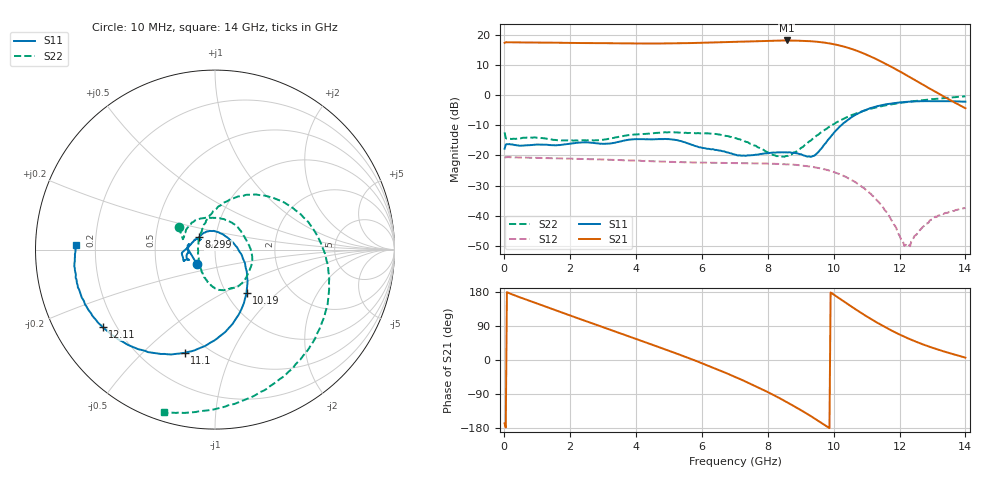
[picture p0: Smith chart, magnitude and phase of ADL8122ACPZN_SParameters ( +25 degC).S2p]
! "Analog Devices, Inc."
! Device:	ADL8122ACPZN
! Description:	"10 kHz to 10 GHz, Wideband, Low Noise Amplifier"
! Conditions:	Vdd = 5.0 V
!		IDQ = 95 mA
!		Pin = -25 dBm
!		Operating Temperature = +25 C (at package bottom)
! Product validation unit SN1 soldered down to Evaluation Board as shown on ADL8122-EVALZ User Guide. Board loss de-embedded from S21 magnitude.  All other RF measurements reference to RF coaxial connector.
! Frequency (GHz)	S11_Mag (dB)	S11_Phase (deg)	S21_Mag (dB)	S21_Phase (deg)	S12_Mag (dB)	S12_Phase (deg)	S22_Mag (dB)	S22_Phase (deg)
#  GHZ  S  DB  R 50
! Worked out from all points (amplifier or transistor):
!   401 points, 10 MHz to 14 GHz, reference 50 ohm
!   highest |S21| = 18.0 dB at 8.579 GHz (marker M1)
!   |S21| within 3 dB of that: start of sweep to 10.6 GHz
!   unconditionally stable (mu >= 1): start of sweep to end of sweep
!   at 2.318 GHz: K = 1.09, MAG = 17.4 dB, |S12| = -21.2 dB
!   at 7.005 GHz: K = 1.12, MAG = 17.9 dB, |S12| = -22.6 dB
!   at 14 GHz: K = 2.02, MAG = 10.7 dB, |S12| = -37.4 dB
!   S11 on the Smith chart (normalised r, x): 10 MHz: 0.81, -0.13; 8.299 GHz: 0.83, +0.12; 10.19 GHz: 1.23, -0.66; 11.1 GHz: 0.38, -0.68; 12.11 GHz: 0.15, -0.31; 14 GHz: 0.13, +0.02
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0.01  -17.82 -141.9  17.25 -167.4  -20.81 12.6  -12.40 147.7
0.184875  -16.37 170.2  17.44 175.0  -20.63 -3.8  -14.54 159.7
1.024275  -16.43 178.5  17.35 148.0  -20.84 -24.8  -14.12 125.2
1.6888  -16.59 -173.4  17.27 127.1  -21.00 -40.9  -15.00 93.4
2.353325  -15.73 -166.2  17.19 106.4  -21.19 -57.1  -15.05 54.8
3.472525  -15.53 -160.6  17.09 71.9  -21.54 -85.5  -13.88 -3.1
4.69665  -14.64 -170.0  17.04 33.9  -22.02 -118.2  -12.53 -46.3
5.920775  -17.33 166.5  17.25 -5.7  -22.38 -152.4  -12.70 -72.8
6.4454  -18.21 152.1  17.41 -23.9  -22.50 -167.8  -12.99 -85.0
7.005  -19.78 145.9  17.60 -44.5  -22.57 175.2  -14.26 -99.4
7.7045  -19.75 148.0  17.84 -72.1  -22.67 152.7  -17.36 -124.6
8.299075  -19.01 141.5  18.01 -98.0  -22.84 132.0  -20.27 -166.6
8.578875  -19.05 129.0  18.04 -111.1  -23.00 121.4  -20.20 164.4
9.348325  -20.34 45.4  17.75 -150.3  -23.83 89.7  -14.65 100.4
9.768025  -15.81 -17.2  17.25 -173.8  -24.75 70.2  -11.34 77.9
10.18772  -10.45 -54.2  16.36 161.7  -26.27 49.4  -8.49 54.6
10.6424  -6.70 -82.9  14.88 135.2  -28.79 26.2  -6.29 29.6
11.09707  -4.44 -106.4  12.86 110.1  -32.50 3.4  -4.67 5.2
11.69165  -2.91 -131.4  9.68 80.7  -40.24 -32.8  -3.20 -24.5
12.11135  -2.37 -145.4  7.16 62.8  -48.76 -87.9  -2.49 -43.2
12.95075  -2.02 -164.7  1.89 33.8  -41.36 152.9  -1.45 -75.9
14  -2.23 178.0  -4.42 6.2  -37.42 123.5  -0.44 -107.3
